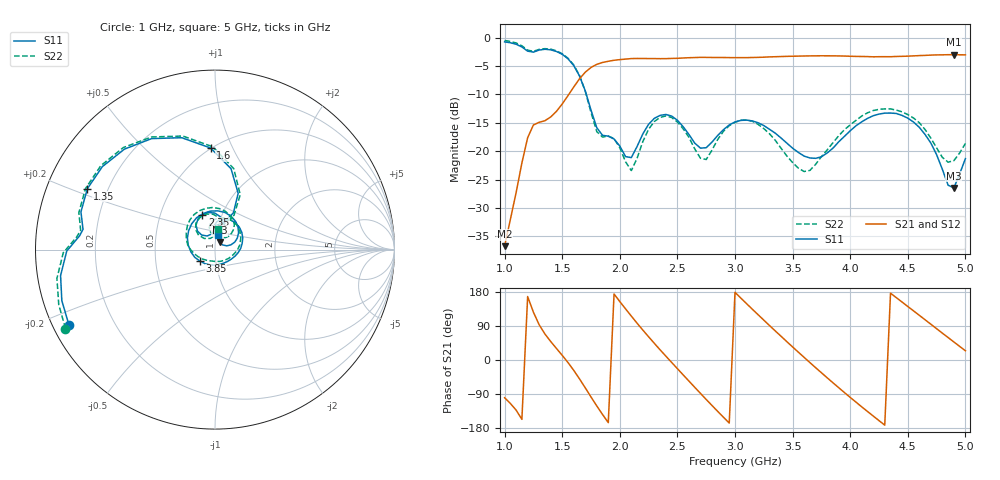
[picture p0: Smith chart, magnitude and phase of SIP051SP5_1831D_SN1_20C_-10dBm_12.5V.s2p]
# GHz  S  dB  R  50
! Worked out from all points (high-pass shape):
!   81 points, 1 GHz to 5 GHz, reference 50 ohm
!   highest |S21| = -3.03 dB at 4.9 GHz (marker M1); lowest = -36.7 dB at 1 GHz (marker M2)
!   |S21| within 3 dB of the highest: 1.705 GHz to end of sweep
!   lowest |S11| = -26.5 dB at 4.9 GHz (marker M3), VSWR 1.10, Z = 52.5 + j4.2 ohm
!   |S11| at or under -10 dB: 1.709 GHz to end of sweep
!   |S22| runs from -23.6 to -0.5 dB; largest |S21 - S12| = 0.0034
!   S11 on the Smith chart (normalised r, x): 1 GHz: 0.05, -0.24; 1.35 GHz: 0.12, +0.22; 1.6 GHz: 0.50, +0.83; 2.35 GHz: 0.81, +0.33; 3.85 GHz: 0.84, -0.11; 5 GHz: 1.02, +0.17
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1  -0.77 -152.8  -36.74 -99.6  -36.83 -99.8  -0.52 -152.2
1.2  -2.40 174.2  -17.64 167.4  -17.61 167.3  -2.23 174.7
1.35  -2.07 154.4  -14.65 68.7  -14.62 68.5  -1.96 154.8
1.6  -4.93 92.5  -8.71 -27.3  -8.71 -27.3  -4.83 91.3
1.7  -9.38 67.6  -6.11 -73.4  -6.12 -73.4  -9.46 65.3
1.8  -15.88 71.0  -4.72 -121.2  -4.73 -121.3  -16.57 70.8
1.95  -17.88 90.5  -4.01 174.2  -4.02 174.3  -17.79 89.2
2.15  -19.18 132.3  -3.69 97.1  -3.69 97.1  -21.27 134.1
2.35  -13.71 109.8  -3.73 26.8  -3.72 26.9  -14.07 115.0
2.5  -14.57 81.5  -3.66 -22.9  -3.65 -22.9  -14.89 83.0
2.7  -19.48 79.3  -3.50 -88.0  -3.51 -88.1  -21.26 79.4
3  -14.86 71.3  -3.54 178.5  -3.53 178.6  -14.94 81.6
3.2  -15.01 32.9  -3.50 119.7  -3.50 119.7  -15.28 36.5
3.35  -16.85 2.9  -3.38 76.6  -3.38 76.7  -18.11 -1.5
3.55  -20.23 -41.5  -3.28 20.7  -3.26 20.5  -22.99 -68.3
3.7  -21.27 -87.8  -3.23 -20.3  -3.23 -20.2  -22.33 -129.7
3.85  -19.49 -142.9  -3.23 -60.0  -3.24 -60.1  -18.53 -169.4
4.05  -15.55 157.3  -3.33 -111.1  -3.32 -111.1  -14.60 149.5
4.35  -13.30 85.9  -3.38 176.4  -3.38 176.4  -12.58 92.9
4.65  -17.07 27.3  -3.15 106.2  -3.14 106.2  -16.21 47.7
4.9  -26.47 57.4  -3.03 47.6  -3.02 47.6  -21.67 71.7
5  -21.33 78.3  -3.05 24.4  -3.06 24.4  -18.66 80.5
